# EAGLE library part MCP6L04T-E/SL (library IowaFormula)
Quad Low-Offset Low-Power OP AMP The OP-11 is pin compatible with the OP-400 , LM148, HA4741, RM4156, and LT1014 operational amplifiers source http://products.analog.com/products/info.asp?product=OP400
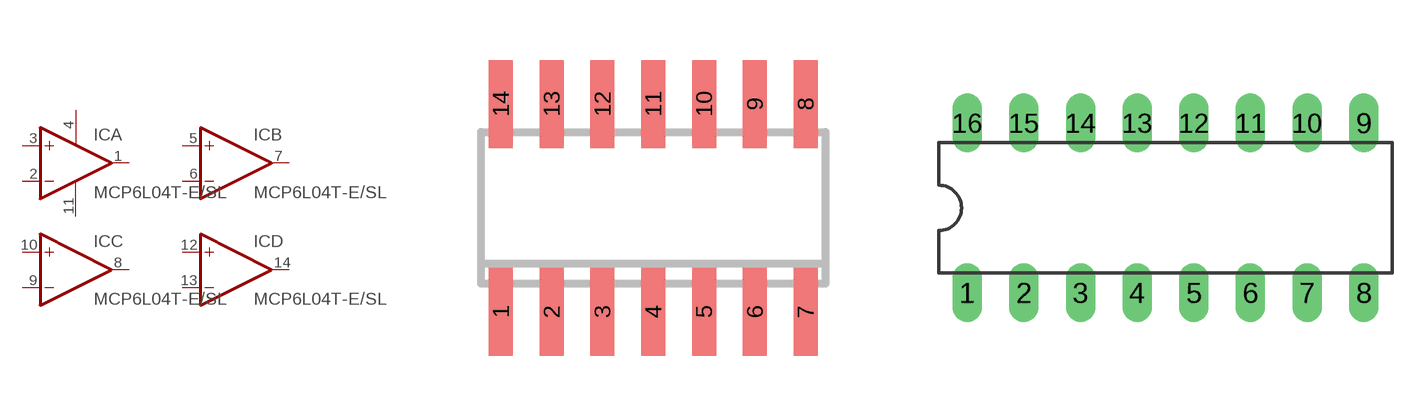
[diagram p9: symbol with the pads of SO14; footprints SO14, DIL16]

Designator prefix IC; gates A=OPAMP B=OPAMP C=OPAMP D=OPAMP P=PWR+-

## MCP6L04T-E/SLD  [SO14]
1  A:OUT  out
2  A:-IN  in
3  A:+IN  in
4  P:V+  pwr
5  B:+IN  in
6  B:-IN  in
7  B:OUT  out
8  C:OUT  out
9  C:-IN  in
10  C:+IN  in
11  P:V-  pwr
12  D:+IN  in
13  D:-IN  in
14  D:OUT  out

## MCP6L04T-E/SLS  [DIL16]
1  A:OUT  out
2  A:-IN  in
3  A:+IN  in
4  P:V+  pwr
5  B:+IN  in
6  B:-IN  in
7  B:OUT  out
10  C:OUT  out
11  C:-IN  in
12  C:+IN  in
13  P:V-  pwr
14  D:+IN  in
15  D:-IN  in
16  D:OUT  out

## MCP6L04T-E/SLTC  [PLCC28S]
2  A:OUT  out
3  A:-IN  in
6  A:+IN  in
8  P:V+  pwr
10  B:+IN  in
13  B:-IN  in
14  B:OUT  out
16  C:OUT  out
17  C:-IN  in
20  C:+IN  in
22  P:V-  pwr
24  D:+IN  in
27  D:-IN  in
28  D:OUT  out

## MCP6L04T-E/SLP  [DIL14]
Pads as for SO14

## Footprint SO14 (pad centres in mm)
Small Outline Package 14
smd 0.6 x 2.2: 1 -3.81,-2.6; 2 -2.54,-2.6; 3 -1.27,-2.6; 4 0,-2.6; 5 1.27,-2.6; 6 2.54,-2.6; 7 3.81,-2.6; 8 3.81,2.6; 9 2.54,2.6; 10 1.27,2.6; 11 0,2.6; 12 -1.27,2.6; 13 -2.54,2.6; 14 -3.81,2.6

## Footprint DIL16 (pad centres in mm)
Dual In Line Package
drill 0.813 long: 1 -8.89,-3.81; 2 -6.35,-3.81; 3 -3.81,-3.81; 4 -1.27,-3.81; 5 1.27,-3.81; 6 3.81,-3.81; 7 6.35,-3.81; 8 8.89,-3.81; 9 8.89,3.81; 10 6.35,3.81; 11 3.81,3.81; 12 1.27,3.81; 13 -1.27,3.81; 14 -3.81,3.81; 15 -6.35,3.81; 16 -8.89,3.81

## Footprint PLCC28S (pad centres in mm)
PLASTIC LEADED CHIP CARRIER square
smd 0.6 x 2.2: 1 0,5.6; 2 -1.27,5.6; 3 -2.54,5.6; 4 -3.81,5.6; 12 -3.81,-5.6; 13 -2.54,-5.6; 14 -1.27,-5.6; 15 0,-5.6; 16 1.27,-5.6; 17 2.54,-5.6; 18 3.81,-5.6; 26 3.81,5.6; 27 2.54,5.6; 28 1.27,5.6
smd 2.2 x 0.6: 5 -5.6,3.81; 6 -5.6,2.54; 7 -5.6,1.27; 8 -5.6,0; 9 -5.6,-1.27; 10 -5.6,-2.54; 11 -5.6,-3.81; 19 5.6,-3.81; 20 5.6,-2.54; 21 5.6,-1.27; 22 5.6,0; 23 5.6,1.27; 24 5.6,2.54; 25 5.6,3.81

## Footprint DIL14 (pad centres in mm)
Dual In Line Package
drill 0.813 long: 1 -7.62,-3.81; 2 -5.08,-3.81; 3 -2.54,-3.81; 4 0,-3.81; 5 2.54,-3.81; 6 5.08,-3.81; 7 7.62,-3.81; 8 7.62,3.81; 9 5.08,3.81; 10 2.54,3.81; 11 0,3.81; 12 -2.54,3.81; 13 -5.08,3.81; 14 -7.62,3.81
